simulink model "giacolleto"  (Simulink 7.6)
settings: Solver=ode14x  StartTime=0.0  StopTime=2e-8  MaxStep=0.001  MinStep=0.0001  RelTol=1e-3
StopFcn:
  | delete *.mat
libraries: fl_lib x10, nesl_utility x3, AppliElectrical_lib x1

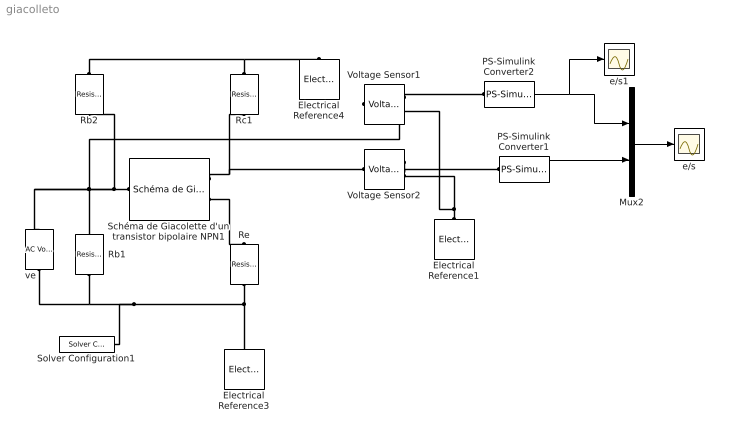
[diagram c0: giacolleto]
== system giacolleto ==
  Electrical Reference1 : fl_lib/Electrical/Electrical Elements/Electrical Reference  DialogController=NetworkEngine.DynNeDlgSource  SystemSampleTime=-1  i_Log=off  LocalVarNames=|i  LocalVarDescs=|i  LocalVarLogging=0
  Electrical Reference3 : fl_lib/Electrical/Electrical Elements/Electrical Reference  DialogController=NetworkEngine.DynNeDlgSource  SystemSampleTime=-1  i_Log=off  LocalVarNames=|i  LocalVarDescs=|i  LocalVarLogging=0
  Electrical Reference4 : fl_lib/Electrical/Electrical Elements/Electrical Reference  DialogController=NetworkEngine.DynNeDlgSource  SystemSampleTime=-1  i_Log=off  LocalVarNames=|i  LocalVarDescs=|i  LocalVarLogging=0
  Mux2 : Mux  Inputs=2
  PS-Simulink Converter1 : nesl_utility/PS-Simulink Converter  DialogController=NetworkEngine.DynNeUtilDlgSource  SystemSampleTime=-1  PhysicalDomain=network_engine_domain  LeftPortType=input  RightPortType=output  SubClassName=ps_output  Unit=1  AffineConversion=off
  PS-Simulink Converter2 : nesl_utility/PS-Simulink Converter  DialogController=NetworkEngine.DynNeUtilDlgSource  SystemSampleTime=-1  PhysicalDomain=network_engine_domain  LeftPortType=input  RightPortType=output  SubClassName=ps_output  Unit=1  AffineConversion=off
  Rb1 : fl_lib/Electrical/Electrical Elements/Resistor  DialogController=NetworkEngine.DynNeDlgSource  SystemSampleTime=-1  R=12 kOhm  i_Log=off  v_Log=off  LocalVarNames=|i|v  LocalVarDescs=|i|v  LocalVarLogging=[0 0]
  Rb2 : fl_lib/Electrical/Electrical Elements/Resistor  DialogController=NetworkEngine.DynNeDlgSource  SystemSampleTime=-1  R=12 kOhm  i_Log=off  v_Log=off  LocalVarNames=|i|v  LocalVarDescs=|i|v  LocalVarLogging=[0 0]
  Rc1 : fl_lib/Electrical/Electrical Elements/Resistor  DialogController=NetworkEngine.DynNeDlgSource  SystemSampleTime=-1  R=22 kOhm  i_Log=off  v_Log=off  LocalVarNames=|i|v  LocalVarDescs=|i|v  LocalVarLogging=[0 0]
  Re : fl_lib/Electrical/Electrical Elements/Resistor  DialogController=NetworkEngine.DynNeDlgSource  SystemSampleTime=-1  R=12 kOhm  i_Log=off  v_Log=off  LocalVarNames=|i|v  LocalVarDescs=|i|v  LocalVarLogging=[0 0]
  Schéma de Giacolette d'un transistor bipolaire NPN1 : AppliElectrical_lib/Schéma de Giacolette d'un transistor bipolaire NPN  DialogController=NetworkEngine.DynNeDlgSource  SystemSampleTime=-1  Cbe=8e-11 F  Cbc=1e-11 F  h11=1000 Ohm  rbb=100 Ohm  h21=100  g=1e-5 1/Ohm  vb2e_Log=off  vb2c_Log=off  Ib_Log=off  Vbe_Log=off  Ic_Log=off  Vce_Log=off  LocalVarNames=|vb2e|vb2c|Ib|Vbe|Ic|Vce  LocalVarDescs=|Tension entre la base interne et l'émetteur|Tension entre la base interne et le collecteur|courant d'entrée du transistor|tension, Base-Emetteur|courant Collecteur-Emetteur|tension Collecteur-Emetteur  LocalVarLogging=[0 0 0 0 0 0]
  Solver Configuration1 : nesl_utility/Solver Configuration  DialogController=NetworkEngine.DynNeUtilDlgSource  SystemSampleTime=-1  PhysicalDomain=network_engine_domain  LeftPortType=input  RightPortType=generic  SubClassName=solver  Accelerate=off  Profile=off  ResidualTolerance=1e-9  MaxNonlinIter=3  MaxModeIter=2  DoFixedCost=off  UseLocalSampling=off  DoDC=off  LinearAlgebra=Sparse  LocalSolverSampleTime=.001  LocalSolverChoice=NE_BACKWARD_EULER_ADVANCER  UseLocalSolver=off
  Voltage Sensor1 : fl_lib/Electrical/Electrical Sensors/Voltage Sensor  DialogController=NetworkEngine.DynNeDlgSource  SystemSampleTime=-1  i1_Log=off  v1_Log=off  LocalVarNames=|i1|v1  LocalVarDescs=|i1|v1  LocalVarLogging=[0 0]
  Voltage Sensor2 : fl_lib/Electrical/Electrical Sensors/Voltage Sensor  DialogController=NetworkEngine.DynNeDlgSource  SystemSampleTime=-1  i1_Log=off  v1_Log=off  LocalVarNames=|i1|v1  LocalVarDescs=|i1|v1  LocalVarLogging=[0 0]
  e/s : Scope
  e/s1 : Scope
  ve : fl_lib/Electrical/Electrical Sources/AC Voltage Source  DialogController=NetworkEngine.DynNeDlgSource  SystemSampleTime=-1  amp=1 V  shift=0 rad  omega=100 MHz  i_Log=off  v_Log=off  LocalVarNames=|i|v  LocalVarDescs=|i|v  LocalVarLogging=[0 0]
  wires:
  PS-Simulink Converter1/1 -> Mux2/2
  PS-Simulink Converter2/1 -> Mux2/1, e/s1/1
  Mux2/1 -> e/s/1
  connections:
  ve/RConn1 -- Rb1/LConn1 -- Electrical Reference3/LConn1 -- Re/LConn1 -- Solver Configuration1/RConn1
  Schéma de Giacolette d'un transistor bipolaire NPN1/LConn1 -- Rb2/LConn1 -- Rb1/RConn1 -- ve/LConn1 -- Voltage Sensor1/LConn1
  Electrical Reference1/LConn1 -- Voltage Sensor2/RConn2 -- Voltage Sensor1/RConn2
  Voltage Sensor2/RConn1 -- PS-Simulink Converter1/LConn1
  Schéma de Giacolette d'un transistor bipolaire NPN1/RConn1 -- Voltage Sensor2/LConn1 -- Rc1/LConn1
  Rc1/RConn1 -- Rb2/RConn1 -- Electrical Reference4/LConn1
  Schéma de Giacolette d'un transistor bipolaire NPN1/RConn2 -- Re/RConn1
  Voltage Sensor1/RConn1 -- PS-Simulink Converter2/LConn1
